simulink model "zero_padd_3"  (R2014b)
settings: Solver=ode45  StartTime=0.0  StopTime=100  RelTol=1e-3
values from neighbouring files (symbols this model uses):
  fs = 4000    [abtast_rate_1.m]    (also in ad_test_12.m = ',     num2str(fs),'; ad_test_2.m = ',     num2str(fs),'; ad_test_3.m = ',     num2str(fs),'; DA_wandler_spektr_1.m = 100)
  N = 4*1024    (= 4096)    [ad_test_12.m]    (also in ad_test_2.m; ad_test_3.m; DA_wandler_spektr_1.m = 1000; DA_wandler_spektr_2.m = 1024)
  noise = 2    [leakage_4.m]    (also in zero_padd3.m = 0)
  Ts = 1/fs    (= 0.00025)    [abtast_rate_1.m]    (also in ad_test_12.m = 0.0009765625; ad_test_2.m = 0.00048828125; ad_test_3.m = 0.00048828125; DA_wandler_spektr_1.m = 0.01)
undefined symbols (not defined in the file or in its folder): Fs, get
libraries: dspspect3 x1, dspstat3 x1, simulink x1, dspsnks4 x1, dspsigops x1

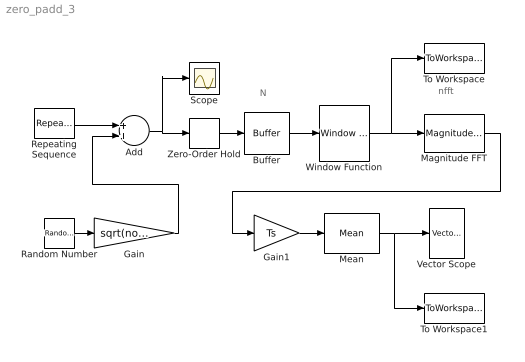
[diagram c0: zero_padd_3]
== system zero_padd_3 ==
  note: nfft
  note: N
  Add : Sum
  Buffer : Buffer  N=N  TreatMby1Signals=One channel
  Gain : Gain  Gain=sqrt(noise)
  Gain1 : Gain  Gain=Ts
  Magnitude FFT : dspspect3/Magnitude FFT  mag_or_magsq=Magnitude  FFTImplementation=Auto  fftLenInherit=off  fftsize=nfft  WrapInput=on
  Mean : dspstat3/Mean  run=on  reset_popup=None  directionMode=Each column  dimension=1  treatSBRowAsCol=on  roiEnable=off  roiType=Rectangles  roiPortion=Entire ROI  roiOutput=Individual statistics for each ROI  roiFlag=off  outputDataTypeStr=Inherit: Same as accumulator  outputLastDataTypeStr=Inherit: Same as accumulator  outputMin=[]  outputMax=[]  roundingMode=Floor  overflowMode=off
  Random Number : RandomNumber  SampleTime=0
  Repeating Sequence : simulink/Sources/Repeating Sequence  rep_seq_t=tsig  rep_seq_y=sig
  Scope : Scope
  To Workspace : ToWorkspace  VariableName=y  SaveFormat=Structure  SampleTime=-1
  To Workspace1 : ToWorkspace  VariableName=Y  SaveFormat=Structure  SampleTime=-1
  Vector Scope : dspsnks4/Vector Scope  ScopeProperties=on  Domain=Frequency  HorizSpan=1  DisplayProperties=off  AxisGrid=on  Memory=off  FrameNumber=on  AxisLegend=off  AxisZoom=off  OpenScopeAtSimStart=on  OpenScopeImmediately=off  FigPos=get(0,'defaultfigureposition')  AxisProperties=off  XUnits=Hertz  XRange=[-Fs/2...Fs/2]  InheritXIncr=off  XIncr=1/1000  XLabel=Time  XLimit=User-defined  XMin=-500  XMax=500  XStart=0  YUnits=Magnitude  YLabel=Amplitude  LineProperties=off  XAxisParamsVer=6.9
  Window Function : dspsigops/Window Function  winmode=Apply window to input  wintype=Boxcar  sampmode=Continuous  samptime=1  N=64  Rs=50  beta=10  winsamp=Symmetric  UserWindow=hamming  OptParams=off  UserParams={'symmetric'}  RowConvenienceOn=on  dataType=double  isSigned=on  wordLen=16  udDataType=sfix(16)  fracBitsMode=Best precision  numFracBits=15  roundingMode=Floor  overflowMode=off  numSidelobes=4  sidelobeLevel=-30
  Zero-Order Hold : ZeroOrderHold  SampleTime=1/fs
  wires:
  Zero-Order Hold/1 -> Buffer/1
  Buffer/1 -> Window Function/1
  Magnitude FFT/1 -> Gain1/1
  Window Function/1 -> Magnitude FFT/1, To Workspace/1
  Gain1/1 -> Mean/1
  Mean/1 -> Vector Scope/1, To Workspace1/1
  Add/1 -> Scope/1, Zero-Order Hold/1
  Repeating Sequence/1 -> Add/1
  Random Number/1 -> Gain/1
  Gain/1 -> Add/2
